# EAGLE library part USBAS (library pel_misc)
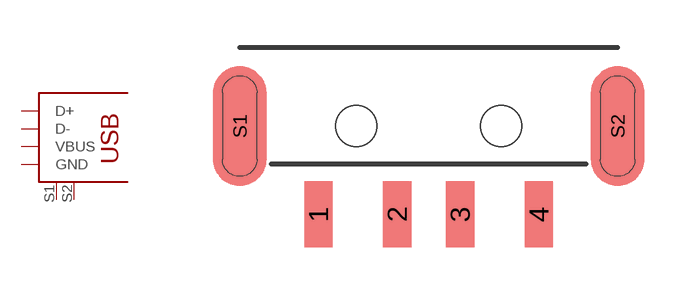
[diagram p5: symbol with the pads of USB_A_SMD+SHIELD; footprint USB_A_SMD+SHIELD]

Designator prefix X

## USBAS-PLUG-SMD  [USB_A_SMD+SHIELD]
1  VBUS
2  D-
3  D+
4  GND
S1  P$1
S2  P$2

## Footprint USB_A_SMD+SHIELD (pad centres in mm)
smd 0.9 x 2.1: 1 -3.5,-2.8; 2 -1,-2.8; 3 1,-2.8; 4 3.5,-2.8
smd 0.635 x 1.27: S1 -6,0; S2 6,0
hole 1.3 at -2.3,0
hole 1.3 at 2.3,0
